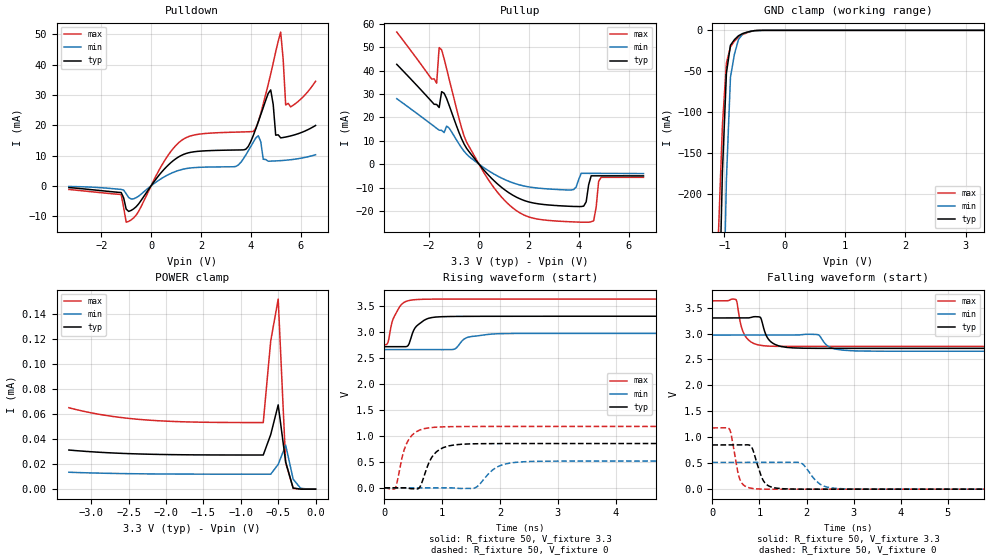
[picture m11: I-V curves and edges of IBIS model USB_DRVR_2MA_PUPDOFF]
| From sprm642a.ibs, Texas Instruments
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|   Model Cell USB_DRVR_2MA_PUPDOFF
|USB_DRVR_2MA_PUPDOFF
[Model]   USB_DRVR_2MA_PUPDOFF
Model_type   I/O
Polarity   Non-Inverting
Enable   Active-Low
Vinl =  0.8
Vinh =  2
Cref =  15.0000pF
Rref =  100.0000M
Vref =  0V
Vmeas =  1.65
C_comp   5.34973p   4.565931p   6.027791p
[Model Spec]
Vinl   0.8   0.8   0.8
Vinh   2   2   2
[Temperature Range]   25   155   -40
[Voltage Range]   3.3   2.97   3.63
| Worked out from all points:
|   slope of the pulldown table from 0 to 0.495 V, typ, clamps not added: 95.1 ohm
|   slope of the pullup table from 0 to 0.495 V, typ, clamps not added: 83.2 ohm
|   GND clamp passes 1 mA (typ) near -0.55 V on its own axis
|   rising waveform, R_fixture 50, V_fixture 3.3: 20-80 % time 190ps typ, 224ps min, 160ps max; typ from 2.71 V to 3.3 V
|   rising waveform, R_fixture 50, V_fixture 0: 20-80 % time 220ps typ, 299ps min, 187ps max; typ from 0 V to 0.852 V
|   falling waveform, R_fixture 50, V_fixture 3.3: 20-80 % time 189ps typ, 222ps min, 168ps max; typ from 3.3 V to 2.71 V
|   falling waveform, R_fixture 50, V_fixture 0: 20-80 % time 192ps typ, 288ps min, 144ps max; typ from 0.852 V to 0 V
| Nom Voltages:
|   BIASFET=3.3, VDD=1.2, VDDS=3.3, VSS=0
| Min Voltages:
|   BIASFET=2.97, VDD=1.08, VDDS=2.97, VSS=0
| Max Voltages:
|   BIASFET=3.63, VDD=1.32, VDDS=3.63, VSS=0
[POWER_clamp]
|   voltage   I(typ)   I(min)   I(max)
-3.3V     31.22uA    13.5uA     64.95uA
-2.8V     29.13uA    12.67uA    58.77uA
-2.3V     27.98uA    12.22uA    55.36uA
-1.7V     27.4uA     12.01uA    53.62uA
-700mV    27.24uA    11.95uA    53.12uA
-600mV    43.52uA    11.94uA    118.2uA
-500mV    67.21uA    19.79uA    151.6uA
-400mV    21.58uA    35.11uA    21.1uA
-300mV    927.4nA    7.959uA    611.4nA
-200mV    28.93nA    716.3nA    11.51nA
0V        696.9pA    39.48nA    568.3pA
[Pulldown]
|   voltage   I(typ)   I(min)   I(max)
-3.3V     -580.7uA   -221.2uA   -1.206mA
-1.2V     -2.224mA   -1.185mA   -2.903mA
-1V       -7.701mA   -2.63mA    -12.01mA
1.2V      9.981mA    5.309mA    14.86mA
3.4V      11.82mA    6.396mA    17.72mA
4.1V      16.62mA    14.41mA    17.95mA
4.3V      21.11mA    16.55mA    21.11mA
4.8V      31.66mA    8.148mA    36.94mA
5V        16.71mA    8.219mA    44.27mA
5.2V      15.82mA    8.317mA    50.76mA
5.4V      16.11mA    8.446mA    26.68mA
6.6V      19.93mA    10.26mA    34.53mA
[Pullup]
|   voltage   I(typ)   I(min)   I(max)
-3.3V     42.67mA    27.99mA    56.47mA
-1.7V     25.52mA    15.35mA    34.62mA
-1.6V     24.22mA    14.55mA    49.83mA
-1.5V     31mA       14.45mA    48.88mA
-500mV    6.805mA    4.314mA    9.445mA
1.6V      -14.6mA    -8.773mA   -20.54mA
3.7V      -18.02mA   -11.02mA   -24.63mA
4.2V      -17.92mA   -3.909mA   -24.78mA
4.5V      -4.967mA   -3.918mA   -24.61mA
4.6V      -4.966mA   -3.921mA   -24.17mA
4.9V      -4.967mA   -3.932mA   -5.627mA
6.6V      -5.001mA   -3.998mA   -5.632mA
[GND_clamp]
|   voltage   I(typ)   I(min)   I(max)
-3.3V     -16.36A    -15.08A    -17.18A
-1.1V     -382.1mA   -717.8mA   -250.1mA
-1.033V   -173.3mA   -402.2mA   -116.4mA
-966.7mV  -52.02mA   -182.1mA   -39.81mA
-900mV    -18.21mA   -57.43mA   -20.34mA
-833.3mV  -11.36mA   -28.88mA   -13.17mA
-766.7mV  -6.618mA   -11.27mA   -8.134mA
-700mV    -3.983mA   -4.59mA    -5.247mA
-500mV    -328.3uA   -481.4uA   -374.5uA
-366.7mV  -15.94uA   -50.74uA   -14.83uA
3.3V      696.9pA    15.85uA    426.1pA
[Ramp]
| variable   typ   min   max
dV/dt_f 0.36646067/0.18656318n  0.1967659/0.22197166n 0.54761634/0.16770422n
dV/dt_r 0.52375749/0.22147225n 0.31724293/0.30230588n 0.72404355/0.18738031n
R_load = 50
[Rising Waveform]
R_fixture = 50
V_fixture = 3.3
V_fixture_min = 2.97
V_fixture_max = 3.63
|   time   V(typ)   V(min)   V(max)
0s        2.714V     2.658V     2.752V
60.9ps    2.714V     2.658V     2.797V
139.9ps   2.714V     2.658V     3.219V
272ps     2.714V     2.658V     3.497V
409ps     2.735V     2.658V     3.598V
610.2ps   3.16V      2.658V     3.624V
1.193ns   3.296V     2.662V     3.629V
1.436ns   3.298V     2.892V     3.63V
2.074ns   3.299V     2.966V     3.63V
20.03ns   3.3V       2.97V      3.63V
[Rising Waveform]
R_fixture = 50
V_fixture = 0
V_fixture_min = 0
V_fixture_max = 0
|   time   V(typ)   V(min)   V(max)
0s        0V         0V         0V
186.9ps   0V         0V         -5.442mV
365.4ps   0V         0V         805.5mV
586.9ps   -15.09mV   0V         1.099V
796.1ps   542.1mV    0V         1.157V
967.6ps   744.6mV    0V         1.171V
1.547ns   847.3mV    -9.339mV   1.18V
1.999ns   851.2mV    425.2mV    1.18V
2.534ns   851.7mV    507.6mV    1.181V
20.01ns   852.2mV    515.3mV    1.181V
[Falling Waveform]
R_fixture = 50
V_fixture = 3.3
V_fixture_min = 2.97
V_fixture_max = 3.63
|   time   V(typ)   V(min)   V(max)
0s        3.3V       2.97V      3.63V
500.2ps   3.3V       2.97V      3.654V
694.7ps   3.3V       2.97V      2.957V
1.017ns   3.314V     2.97V      2.774V
1.161ns   2.933V     2.97V      2.758V
1.471ns   2.749V     2.97V      2.752V
2.236ns   2.715V     2.979V     2.752V
2.54ns    2.714V     2.72V      2.752V
3.235ns   2.714V     2.662V     2.752V
20.03ns   2.714V     2.658V     2.752V
[Falling Waveform]
R_fixture = 50
V_fixture = 0
V_fixture_min = 0
V_fixture_max = 0
|   time   V(typ)   V(min)   V(max)
0s        852.2mV    515.3mV    1.181V
360.5ps   852.1mV    515.3mV    1.16V
597ps     852.2mV    515.3mV    162.9mV
819.8ps   828.6mV    515.3mV    18.14mV
929.3ps   554.5mV    515.3mV    5.642mV
1.144ns   95.51mV    515.2mV    0V
1.529ns   6.865mV    515.3mV    0V
1.873ns   0V         506.7mV    0V
2.772ns   0V         7.893mV    0V
20.01ns   0V         0V         0V
